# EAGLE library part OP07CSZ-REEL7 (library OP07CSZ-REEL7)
Precision Amplifiers Ultra Low Offset VTG Source: Datasheet
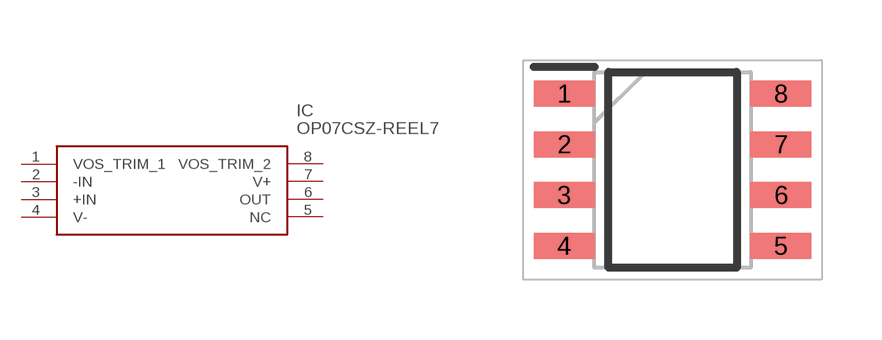
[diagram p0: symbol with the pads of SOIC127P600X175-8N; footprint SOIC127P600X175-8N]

Designator prefix IC

## OP07CSZ-REEL7 (Arrow_Part_Number: OP07CSZ-REEL7; Arrow_Price-Stock: https://www.arrow.com/en/products/op07csz-reel7/analog-devices?region=nac; Description: Precision Amplifiers Ultra Low Offset VTG; Height: 1.75mm; Manufacturer_Name: Analog Devices; Manufacturer_Part_Number: OP07CSZ-REEL7; Mouser_Part_Number: 584-OP07CSZ-R7; Mouser_Price-Stock: https://www.mouser.co.uk/ProductDetail/Analog-Devices/OP07CSZ-REEL7?qs=WIvQP4zGangZT8LGnisnoQ%3D%3D)  [SOIC127P600X175-8N]
1  VOS_TRIM_1
2  -IN  in
3  +IN  in
4  V-
5  NC  nc
6  OUT  out
7  V+
8  VOS_TRIM_2

## Footprint SOIC127P600X175-8N (pad centres in mm)
R-8 (SOIC)
smd 1.525 x 0.65: 1 -2.712,1.905; 2 -2.712,0.635; 3 -2.712,-0.635; 4 -2.712,-1.905; 5 2.712,-1.905; 6 2.712,-0.635; 7 2.712,0.635; 8 2.712,1.905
